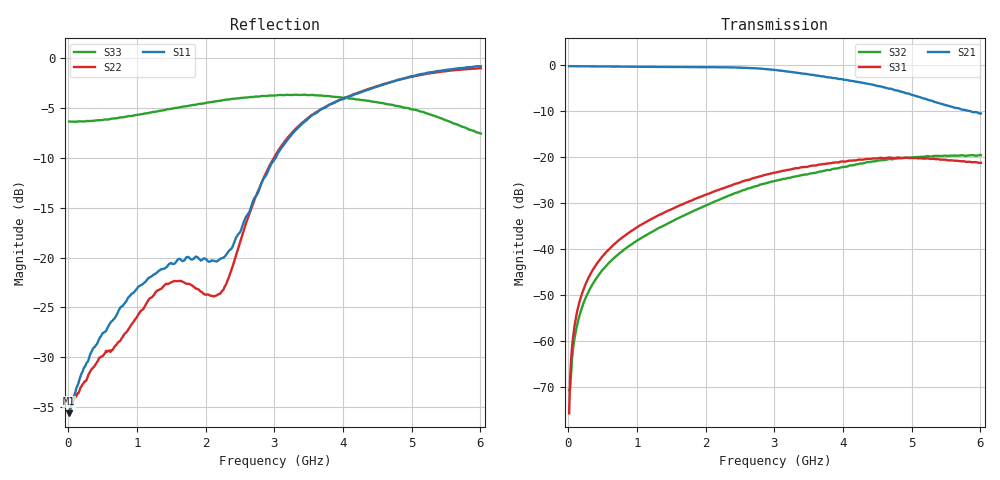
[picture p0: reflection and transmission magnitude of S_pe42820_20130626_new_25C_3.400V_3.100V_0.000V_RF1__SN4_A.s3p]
! Device ID: pe42820_20130626_new
! Dir: c:\SVN\PSC 4Port_VNA Bench\CVI 2009\branches\PE42820\pe42820_matching\pe42820_20130626_new\25C\3p400000\RF1
! Serial: 4
! Insertion: A
! Temp: 25C
! VDD: 3.400
! Control_Hi: 3.100
! Control_Lo: 0.000
! Logic State: RF1
! ThroughPath: 2-1
! Port 1: RFC
! Port 2: RF1
! Port 3: RF2
! V1 = 3.10
! V2 = 0.00
! V3 = 0.00
! IDD: 1.334566e-04
! FILE NAME
! DATE 06/27/13  15:31
! CORRECTED  DATA
#  Hz  S  RI  R  50
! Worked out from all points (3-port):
!   401 points, 10 MHz to 6.01 GHz, reference 50 ohm
!   strongest paths, dB at 10 MHz, 1.51 GHz, 3.01 GHz, 4.51 GHz, 6.01 GHz:
!     S21: -0.2, -0.3, -1.0, -4.5, -10.4
!     S31: -75.7, -31.2, -23.3, -20.2, -21.2
!     S32: -70.7, -33.9, -25.2, -20.7, -19.5
!   lowest |S11| = -35.6 dB at 10 MHz (marker M1), VSWR 1.03, Z = 51.7 + j0.166 ohm
!   |S11| at or under -10 dB: start of sweep to 3.018 GHz
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1e7  0.0164 0.0016  0.9809 -0.00822  8.98e-05 0.000147
     0.9808 -0.00875  0.0168 0.00157  0.000196 0.000121
     5.46e-05 0.000154  0.000229 0.000183  -0.482 0.00652
7e7  0.0188 0.00501  0.9784 -0.057  0.000142 0.00115
     0.9786 -0.0565  0.018 0.00586  0.000116 0.000823
     0.000134 0.00113  0.000128 0.000838  -0.4796 0.0382
1.6e8  0.023 0.00812  0.9705 -0.1273  0.000289 0.00264
       0.9706 -0.1282  0.0187 0.0105  0.000253 0.00186
       0.000304 0.00265  0.000247 0.00187  -0.475 0.0859
5.65e8  0.0435 0.00727  0.8739 -0.4279  0.00292 0.0091
        0.8738 -0.4274  0.0209 0.0264  0.00187 0.00652
        0.00291 0.00908  0.00189 0.0065  -0.4057 0.2799
1.885e9  0.0316 -0.0951  0.0443 -0.9564  0.031 0.0177
         0.0462 -0.9582  0.031 0.062  0.022 0.0161
         0.0315 0.0181  0.0221 0.0162  0.0979 0.5803
2.275e9  -0.0634 -0.0785  -0.2718 -0.9156  0.0451 0.012
         -0.2737 -0.9126  -0.0148 0.0696  0.0338 0.0136
         0.0452 0.0116  0.034 0.0136  0.2396 0.5691
3.01e9  -0.2001 0.2401  -0.7384 -0.4978  0.0647 -0.0231
        -0.7403 -0.4979  -0.1525 0.2852  0.0545 -0.0119
        0.0642 -0.0228  0.0539 -0.0118  0.4462 0.4738
4.06e9  0.3483 0.5352  -0.655 0.2228  0.0299 -0.0855
        -0.6579 0.2223  0.0979 0.632  0.0414 -0.0677
        0.0306 -0.0853  0.0418 -0.0675  0.5922 0.2209
4.96e9  0.8038 0.0629  -0.232 0.4277  -0.0427 -0.0882
        -0.2336 0.4338  0.5456 0.5884  -0.0209 -0.0973
        -0.0431 -0.0881  -0.0207 -0.0968  0.5608 -0.00285
6.01e9  0.7921 -0.4502  0.0078 0.299  -0.0828 -0.0277
        0.00434 0.3005  0.8328 0.3198  -0.0901 -0.0564
        -0.0825 -0.0281  -0.0899 -0.0553  0.415 -0.0593
